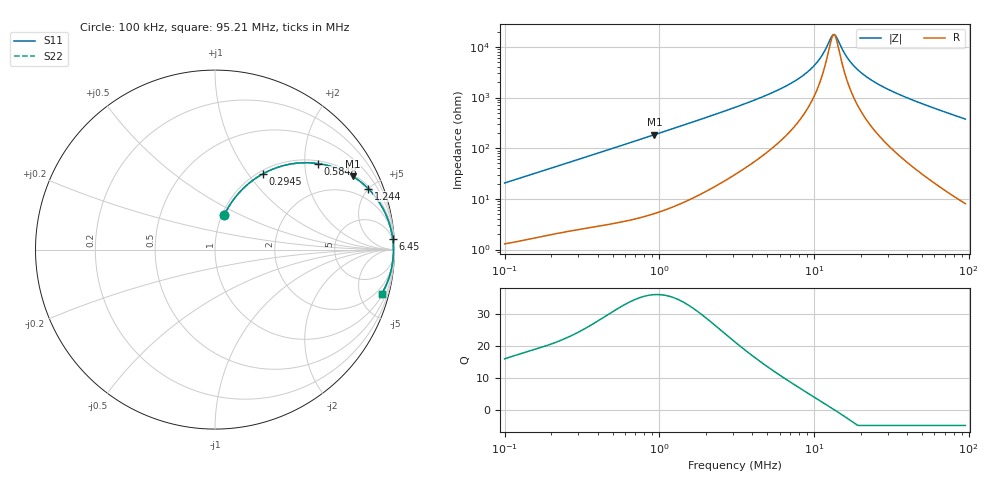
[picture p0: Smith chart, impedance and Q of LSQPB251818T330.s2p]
! LSQPB251818T330  S-PARAMETER MODEL  ( General Type )
! Model Generated by TAIYO YUDEN Corporation (http://www.ty-top.com)
! Version 2.0
! TAIYO YUDEN Control No. 100810NG19SB-FKC
! Copyright(c) 2009 TAIYO YUDEN CO.,LTD. All Rights Reserved.
! Product Description (link to TY-COMPAS)
! https://ds.yuden.co.jp/TYCOMPAS/or/detail?pn=LSQPB251818T330K&u=M
! Products Name : Inductors
! Characteristics :
!  Inductance : 33 uH , SRF(min) : 8.0 MHz , DC Resistance(max) : 1.105 Ohm
!  Rated Current : Saturation :560 mA , Temp Rise : 390 mA (40 degC)
!  Case Size : 2.5 x 1.8 / 0.098 x 0.071 [mm/inch] , Thickness : 1.8 / 0.071 [mm/inch]
!  (Conditions: Temperature = 25 degC , DC Bias Current/Voltage = 0A / 0V)
! External Node Assignments :
!  1  o---GGG---o  2
! GND o---------o GND
! Frequency Range : 0.1MHz  -  95.211795MHz  [ 402 STEP ]
# MHz S RI R 50
! Freq[MHz].  S11 Real  S11 Imag  S21 Real  S21 Imag  S12 Real  S12 Imag  S22 Real  S22 Imag
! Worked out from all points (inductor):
!   401 points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, 100 kHz to 95.21 MHz, reference 50 ohm
!   read as one part in series: L = 32.5 uH near 103.5 kHz
!   highest Q = 36.1 at 929.1 kHz (marker M1), where L = 31.6 uH
!   self-resonance near 13.25 MHz
!   S11 on the Smith chart (normalised r, x): 100 kHz: 1.03, +0.41; 294.5 kHz: 1.05, +1.18; 584.8 kHz: 1.07, +2.32; 1.244 MHz: 1.14, +4.95; 6.45 MHz: 4, +32; 95.21 MHz: 1.16, -7.52
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0.1  0.0517 0.1921  0.9483 -0.1921  0.9483 -0.1921  0.0517 0.1921
0.179138  0.1288 0.3106  0.8712 -0.3106  0.8712 -0.3106  0.1288 0.3106
0.29454  0.2671 0.4222  0.7329 -0.4222  0.7329 -0.4222  0.2671 0.4222
0.31545  0.2928 0.4354  0.7072 -0.4354  0.7072 -0.4354  0.2928 0.4354
0.584807  0.5723 0.4797  0.4277 -0.4797  0.4277 -0.4797  0.5723 0.4797
0.929126  0.7668 0.4093  0.2332 -0.4093  0.2332 -0.4093  0.7668 0.4093
0.995088  0.7898 0.3938  0.2102 -0.3938  0.2102 -0.3938  0.7898 0.3938
1.243566  0.8527 0.3404  0.1473 -0.3404  0.1473 -0.3404  0.8527 0.3404
3.085641  0.9694 0.1502  0.0306 -0.1502  0.0306 -0.1502  0.9694 0.1502
6.449925  0.9902 0.06  0.00983 -0.06  0.00983 -0.06  0.9902 0.06
8.199905  0.9925 0.0387  0.00747 -0.0387  0.00747 -0.0387  0.9925 0.0387
9.733658  0.9936 0.0247  0.00645 -0.0247  0.00645 -0.0247  0.9936 0.0247
10.97497  0.994 0.0154  0.00599 -0.0154  0.00599 -0.0154  0.994 0.0154
12.8063  0.9943 0.00367  0.00568 -0.00367  0.00568 -0.00367  0.9943 0.00367
13.4823  0.9944 -0.000206  0.00564 0.000206  0.00564 0.000206  0.9944 -0.000206
14.19398  0.9944 -0.00409  0.00564 0.00409  0.00564 0.00409  0.9944 -0.00409
16.28088  0.9942 -0.0145  0.00578 0.0145  0.00578 0.0145  0.9942 -0.0145
18.67462  0.9938 -0.0252  0.00616 0.0252  0.00616 0.0252  0.9938 -0.0252
22.941  0.9927 -0.0423  0.00725 0.0423  0.00725 0.0423  0.9927 -0.0423
30.70484  0.9897 -0.0695  0.0103 0.0695  0.0103 0.0695  0.9897 -0.0695
50.48494  0.9774 -0.1298  0.0226 0.1298  0.0226 0.1298  0.9774 -0.1298
95.21179  0.9293 -0.2458  0.0707 0.2458  0.0707 0.2458  0.9293 -0.2458
